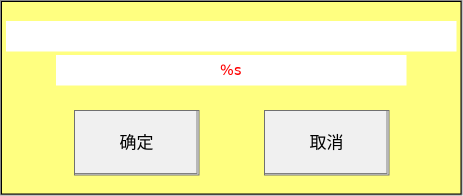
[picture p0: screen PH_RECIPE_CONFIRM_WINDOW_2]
VISUALIZATION PH_RECIPE_CONFIRM_WINDOW_2  // 463x196
VAR_IN_OUT
	RECIPE_CTRL_V2 : ST_RecipeCtrl_2;
END_VAR
    Group (1,1 460x193), invisible if: NOT RECIPE_CTRL_V2.sStatus.bShowDialog
        Rectangle (0,0 460x193), colour toggle: (RECIPE_CTRL_V2.sStatus.bFlashLamp) <> 0
        Rectangle (5,20 450x30), text list: 'question', text index: RECIPE_CTRL_V2.sStatus.i16ShowDiagID
            p2738717112: SEL(RECIPE_CTRL_V2.sStatus.sgShowDialogMassage = '', 0, 20)
        Rectangle (55,54 350x30), "%s", text variable: RECIPE_CTRL_V2.sStatus.sgShowDialogMassage, invisible if: RECIPE_CTRL_V2.sStatus.sgShowDialogMassage = ''
        Button (73,109 125x65), "确定", text list: 'TextList_Recipe', text index: 120
            p55702900: SEL(RECIPE_CTRL_V2.sCmd.bRecipeConfirmYes, 16#000000, 16#00FF00)
            tap RECIPE_CTRL_V2.sCmd.bRecipeConfirmYes
        Button (263,109 125x65), "取消", text list: 'TextList_Recipe', text index: 121
            p55702900: SEL(RECIPE_CTRL_V2.sCmd.bRecipeConfirmNo, 16#000000, 16#00FF00)
            tap RECIPE_CTRL_V2.sCmd.bRecipeConfirmNo
END_VISUALIZATION
